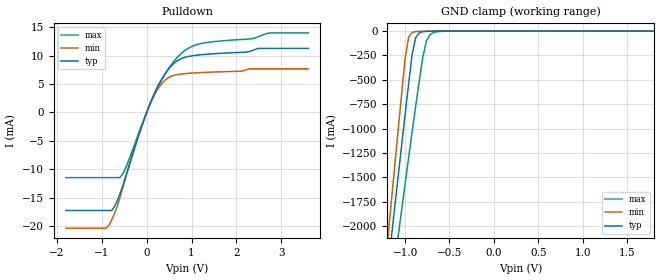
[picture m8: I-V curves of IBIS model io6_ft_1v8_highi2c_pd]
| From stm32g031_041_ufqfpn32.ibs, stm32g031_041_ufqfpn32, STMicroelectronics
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|   Model io6_ft_1v8_highi2c_pd
[Model]  io6_ft_1v8_highi2c_pd
Model_type I/O_open_drain
Polarity   Non-Inverting
Enable   Active-Low
Vinl =   0.540000V
Vinh =   1.260000V
Vmeas =  0.90000V
Cref =   50.000000pF
Rref =   500
Vref =   3.0V
C_comp   1.277600pF   1.236700pF   1.315100pF
[Temperature Range]   25.000000   -40.000000   0.125000k
[Pullup Reference]   1.800000V   1.600000V   2.000000V
[Pulldown Reference]   0.0V   0.0V   0.0V
[POWER Clamp Reference]   1.800000V   1.600000V   2.000000V
[GND Clamp Reference]   0.0V   0.0V   0.0V
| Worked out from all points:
|   slope of the pulldown table from 0 to 0.27 V, typ, clamps not added: 54.7 ohm
|   GND clamp passes 1 mA (typ) near -0.66 V on its own axis
[Pulldown]
|Voltage   I(typ)   I(min)   I(max)
-1.8V     -17.22mA   -20.33mA   -11.45mA
-900mV    -17.22mA   -20.33mA   -11.45mA
-720mV    -16.58mA   -17.82mA   -11.45mA
-600mV    -14.41mA   -15.08mA   -11.45mA
-480mV    -11.58mA   -11.79mA   -9.954mA
0V        10fA       0A         100fA
240mV     4.49mA     3.999mA    4.291mA
480mV     7.563mA    6.085mA    7.612mA
780mV     9.487mA    6.76mA     10.43mA
1.14V     10.08mA    6.976mA    11.96mA
2.76V     11.26mA    7.652mA    13.98mA
3.6V      11.26mA    7.652mA    13.98mA
[GND_clamp]
|Voltage   I(typ)   I(min)   I(max)
-1.8V     -7.471A    -7.973A    -7.298A
-1.2V     -2.489A    -2.18A     -2.954A
-1.16V    -2.16A     -1.797A    -2.674A
-1.08V    -1.505A    -1.034A    -2.118A
-1V       -858mA     -283.1mA   -1.568A
-960mV    -540.4mA   -62.15mA   -1.296A
-920mV    -234.4mA   -13.76mA   -1.028A
-880mV    -66.3mA    -4.868mA   -765.3mA
-800mV    -6.518mA   -2.068mA   -266mA
-760mV    -3.087mA   -1.462mA   -100.4mA
-680mV    -1.228mA   -569.1uA   -14.21mA
1.8V      47.47uA    34.04uA    59.57uA
[POWER_clamp]
|Voltage   I(typ)   I(min)   I(max)
-1.8V     0A         0A         0A
0V        0A         0A         0A
[Ramp]
| variable   typ   min   max
dV/dt_r  0.305/1.74885n   0.210/1.41505n   0.369/1.86730n
dV/dt_f  0.30096/1.46389n   0.210/1.35405n   0.36720/1.46921n
R_load = 50.000000
